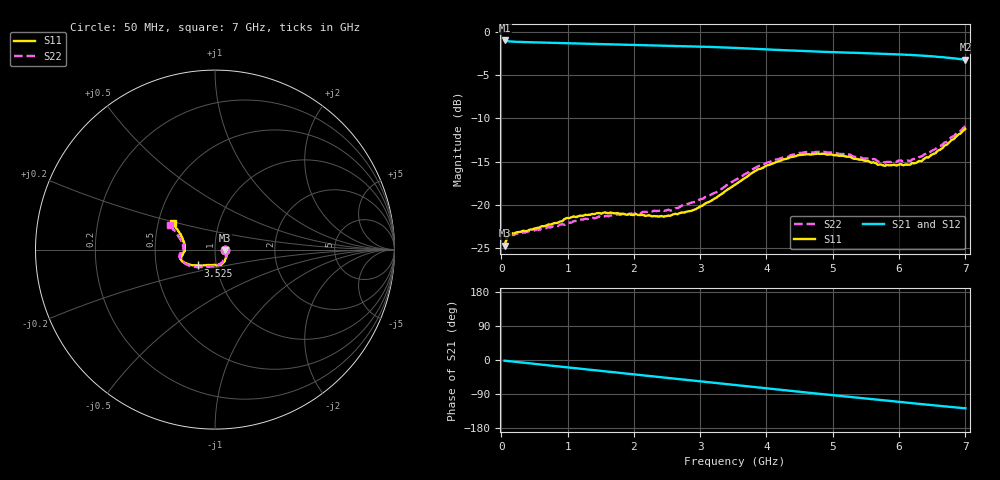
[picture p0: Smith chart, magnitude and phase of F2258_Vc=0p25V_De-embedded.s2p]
! Integrated Device Technology
! Corporate Headquarters
! 6024 Silver Creek Valley Road
! San Jose, CA 95138  USA
! Phone:  1-408-284-8200
! Toll Free:  1-800-223-1366
! Webpage:  http://www.idt.com/
! Timing and RF Division
! 515 Groton Road, Suite 102
! Westford, MA 01886-6024
! Device:  F2258
! Description: Voltage Variable RF Attenuator
! Frequency:  50.0 -  6000.00 MHz
! Package:  3x3 mm Thin QFN Plastic Package: 16 pin
! Ports:  2 RF, 2 DC
!  Pin  1  = NC
!  Pin  2  = NC
!  Pin  3  = RF2  = Port 2
!  Pin  4  = GND
!  Pin  5  = Vdd
!  Pin  6  = NC
!  Pin  7  = VCTRL
!  Pin  8  = NC
!  Pin  9  = GND
!  Pin 10  = RF1  = Port 1
!  Pin 11  = NC
!  Pin 12  = NC
!  Pin 13  = NC
!  Pin 14  = NC
!  Pin 15  = NC
!  Pin 16  = NC
! Vcntrl:  0.250 Volts
! Vdd:  +3.300 Volts
! Current:  1.080 mA
! Data:  The device was measured on a the F2258 evaluation board which has
!  individual transmission lines to the RF pins.  Data was collected
!  using a calibrated network analyzer.  The evaluation board was
!  de-embedded using a TRL calibration technique.
!  The reference plane is the edge of the package pin.
! Misc:  SN 10
!  Action Tracker AT0285
! Date Measured:  2014-12-10
! Date:  2016-01-13  MJV
! Note:
!  Integrated Device Technology supplies this data as a sample of measured
!  data at the package pin for this product.  Your particular data for this
!  product may vary.
!  Data was taken at 25 degrees C.
!  Integrated Device Technology reserves the right to change this data at anytime.
!Freq_(GHz)  S11M_(dB)  S11P_(deg)  S21M_(dB)  S21P_(deg)  S12M_(dB)  S12P_(deg)  S22M_(dB)  S22P_(deg)
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# GHz S dB R 50
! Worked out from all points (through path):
!   201 points, 50 MHz to 7 GHz, reference 50 ohm
!   highest |S21| = -0.96 dB at 50 MHz (marker M1); lowest = -3.2 dB at 7 GHz (marker M2)
!   group delay of S21, straight-line fit = 50.5 ps
!   lowest |S11| = -24.8 dB at 50 MHz (marker M3), VSWR 1.12, Z = 56.1 - j0.394 ohm
!   |S11| at or under -10 dB: start of sweep to end of sweep
!   |S22| runs from -24.8 to -10.9 dB; largest |S21 - S12| = 0.00034
!   S11 on the Smith chart (normalised r, x): 50 MHz: 1.12, -0.01; 3.525 GHz: 0.81, -0.15; 7 GHz: 0.60, +0.19
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0.05  -24.76 -3.5  -0.96 -1.9  -0.96 -1.9  -24.80 -3.0
0.08475  -23.80 -5.9  -1.04 -2.5  -1.04 -2.5  -23.86 -5.4
0.15425  -23.31 -9.2  -1.09 -3.6  -1.09 -3.6  -23.48 -9.4
0.71025  -22.30 -36.8  -1.23 -14.1  -1.22 -14.1  -22.60 -38.4
0.98825  -21.54 -50.6  -1.28 -19.3  -1.28 -19.3  -22.10 -54.5
1.2315  -21.29 -58.9  -1.33 -23.8  -1.33 -23.8  -21.73 -63.5
1.6485  -20.89 -70.6  -1.42 -31.4  -1.42 -31.4  -21.24 -76.5
2.37825  -21.37 -91.9  -1.55 -44.8  -1.55 -44.8  -20.71 -94.1
2.552  -21.28 -97.8  -1.58 -48.0  -1.58 -48.0  -20.67 -99.4
2.93425  -20.52 -114.6  -1.66 -55.1  -1.66 -55.1  -19.68 -112.8
3.525  -17.70 -137.4  -1.83 -66.2  -1.82 -66.2  -17.18 -135.5
4.0115  -15.44 -151.1  -2.01 -75.2  -2.01 -75.2  -15.10 -150.9
4.46325  -14.29 -159.5  -2.17 -83.4  -2.17 -83.4  -14.05 -162.0
4.7065  -14.16 -162.8  -2.24 -87.7  -2.24 -87.7  -13.94 -166.2
5.15825  -14.32 -168.2  -2.36 -95.6  -2.36 -95.6  -14.12 -173.1
5.64475  -15.17 -176.4  -2.48 -104.0  -2.48 -104.0  -14.75 -179.4
5.6795  -15.36 -176.5  -2.47 -104.6  -2.47 -104.6  -15.00 -179.7
5.85325  -15.43 179.3  -2.53 -107.8  -2.53 -107.8  -15.04 175.7
6.166  -15.36 171.5  -2.64 -113.4  -2.64 -113.4  -14.95 169.8
6.33975  -14.95 165.2  -2.72 -116.5  -2.72 -116.5  -14.41 165.4
6.722  -13.03 153.5  -2.95 -123.1  -2.95 -123.1  -12.70 156.4
7  -11.21 148.1  -3.20 -127.4  -3.20 -127.4  -10.91 151.5
